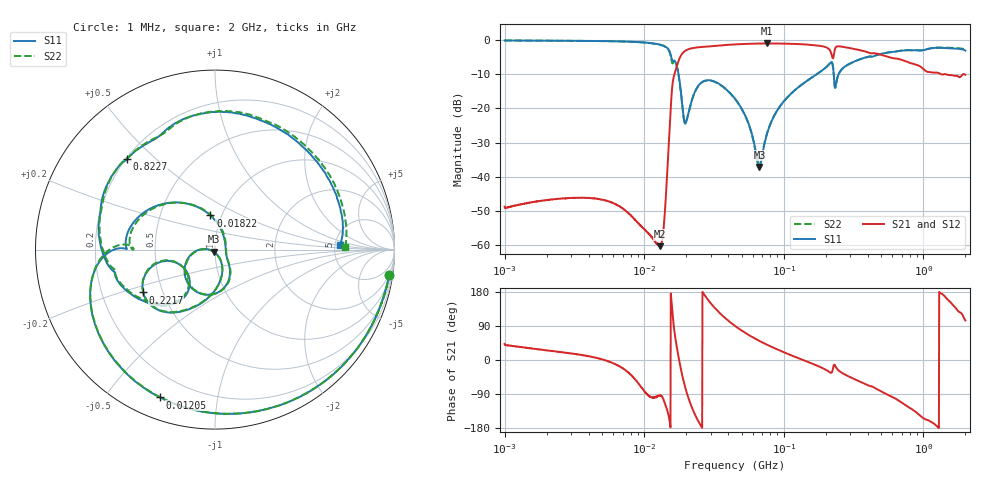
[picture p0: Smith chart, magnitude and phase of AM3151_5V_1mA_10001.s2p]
! Date/Time: Fri Jun 26 10:52:17 2020
! Network Analyzer:  Rev:
! Sweep from 1000000.0 to 2000000000.0, 1601 Points ! Power Supply: 0 V, 0 A
# HZ S DB R 50
!freq MagS11 AngS11 MagS21 AngS21 MagS12 AngS12 MagS22 AngS22
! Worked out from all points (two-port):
!   1601 points, 1 MHz to 2 GHz, reference 50 ohm
!   highest |S21| = -1.04 dB at 75.42 MHz (marker M1); lowest = -60.2 dB at 12.88 MHz (marker M2)
!   |S21| within 3 dB of the highest: 18.69 MHz to 219.2 MHz (200.5 MHz wide, 169 % of centre); 229.1 MHz to 467.4 MHz (238.3 MHz wide, 68.4 % of centre)
!   lowest |S11| = -37.1 dB at 66.97 MHz (marker M3), VSWR 1.03, Z = 49.3 - j1.2 ohm
!   |S11| at or under -10 dB: 17.62 MHz to 172.3 MHz (154.7 MHz wide, 163 % of centre); 227.9 MHz to 247.1 MHz (19.24 MHz wide, 8.1 % of centre)
!   |S22| runs from -37.0 to -0.2 dB; largest |S21 - S12| = 0.0072
!   S11 on the Smith chart (normalised r, x): 1 MHz: 2, -13; 12.05 MHz: 0.10, -0.69; 18.22 MHz: 0.89, +0.35; 221.7 MHz: 0.39, -0.24; 822.7 MHz: 0.20, +0.41; 2 GHz: 5.55, +0.52
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1000000  -0.17 -8.4  -48.70 42.7  -49.08 39.4  -0.17 -8.4
3555161  -0.28 -28.7  -46.12 13.2  -46.09 13.4  -0.27 -28.8
7147290  -0.47 -59.0  -49.51 -24.2  -49.45 -24.1  -0.48 -59.2
1.205276e7  -1.13 -110.4  -58.97 -96.9  -59.05 -98.9  -1.15 -111.2
1.263916e7  -1.28 -118.5  -59.92 -95.0  -59.98 -94.6  -1.31 -119.4
1.288164e7  -1.35 -122.1  -60.23 -93.1  -60.32 -93.4  -1.39 -123.0
1.389893e7  -1.78 -139.1  -53.24 -109.3  -53.16 -108.9  -1.84 -140.5
1.602785e7  -6.18 179.6  -12.26 115.9  -12.24 115.8  -6.85 -180.0
1.822133e7  -14.34 97.6  -4.75 -19.8  -4.75 -19.8  -14.54 94.9
1.947442e7  -24.22 18.4  -3.32 -66.4  -3.31 -66.4  -24.00 14.4
2.071503e7  -21.46 -36.6  -2.72 -99.7  -2.73 -99.7  -21.48 -36.1
2.553075e7  -12.54 -84.4  -2.07 -174.1  -2.07 -174.1  -12.60 -82.6
3.33119e7  -12.51 -131.3  -1.71 130.8  -1.70 130.8  -12.57 -130.0
4.493426e7  -17.29 -168.2  -1.31 89.4  -1.30 89.4  -17.36 -167.2
6.697021e7  -37.09 -119.5  -1.06 50.2  -1.07 50.2  -36.94 -115.3
7.541541e7  -27.75 -63.4  -1.04 40.7  -1.04 40.7  -27.59 -62.9
1.589914e8  -10.96 -100.2  -1.48 -9.3  -1.47 -9.3  -10.98 -100.5
2.217143e8  -6.61 -149.2  -4.78 -31.6  -4.80 -31.6  -6.65 -149.6
5.652395e8  -3.66 170.6  -5.01 -93.1  -4.99 -93.1  -3.67 168.6
8.226611e8  -3.06 134.3  -6.85 -129.0  -6.80 -128.9  -3.04 131.7
1.322926e9  -2.29 77.6  -9.93 176.9  -9.85 176.5  -2.21 74.9
2e9  -3.13 2.0  -10.19 104.4  -10.34 103.8  -2.78 1.0
